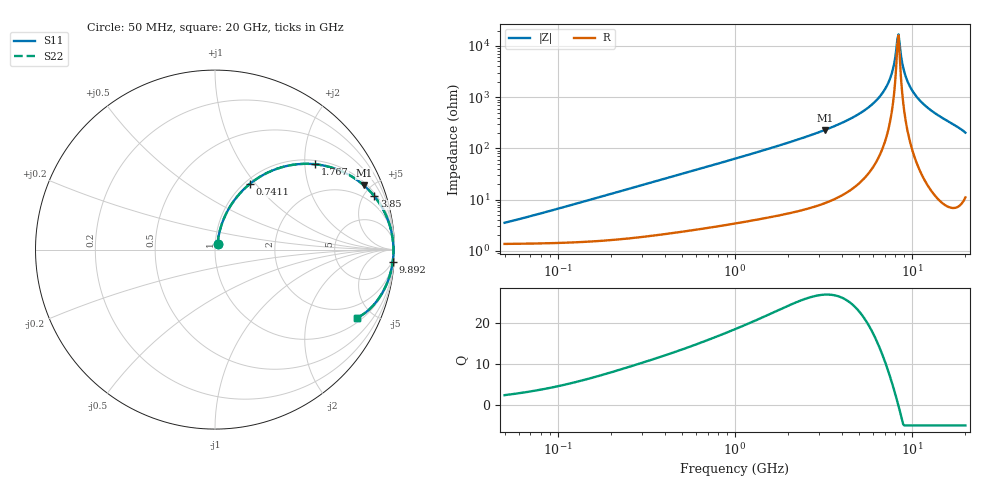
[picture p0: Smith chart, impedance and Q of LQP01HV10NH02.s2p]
!Murata Part Number: LQP01HV10NH02
!These Parameters are Measured in Series Mode Connection
!  o--[Z]--o
!Port1  Port2
!  o-------o
!Freq. Start=50[MHz] Stop=20[GHz], 401[Steps]
# Hz S RI R 50
!Freq.(Hz) S11(Real) S11(Imag) S21(Real) S21(Imag) S12(Real) S12(Imag) S22(Real) S22(Imag)
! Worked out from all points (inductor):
!   401 points, 50 MHz to 20 GHz, reference 50 ohm
!   read as one part in series: L = 10.3 nH near 63.54 MHz
!   highest Q = 26.9 at 3.217 GHz (marker M1), where L = 11.3 nH
!   self-resonance near 8.265 GHz
!   S11 on the Smith chart (normalised r, x): 50 MHz: 1.03, +0.06; 741.1 MHz: 1.06, +0.93; 1.767 GHz: 1.10, +2.26; 3.85 GHz: 1.22, +5.90; 9.892 GHz: 3, -29; 20 GHz: 1.22, -4.05
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5e7  0.0144 0.0315  0.9856 -0.0315  0.9856 -0.0315  0.0144 0.0315
1.364002e8  0.0219 0.0848  0.9781 -0.0848  0.9781 -0.0848  0.0219 0.0848
3.721004e8  0.0699 0.2155  0.9301 -0.2155  0.9301 -0.2155  0.0699 0.2155
7.411344e8  0.1931 0.3651  0.8069 -0.3651  0.8069 -0.3651  0.1931 0.3651
1e9  0.2932 0.4289  0.7068 -0.4289  0.7068 -0.4289  0.2932 0.4289
1.766834e9  0.5587 0.4754  0.4413 -0.4754  0.4413 -0.4754  0.5587 0.4754
2.728004e9  0.766 0.4049  0.234 -0.4049  0.234 -0.4049  0.766 0.4049
3.216634e9  0.8303 0.3572  0.1697 -0.3572  0.1697 -0.3572  0.8303 0.3572
3.850025e9  0.8881 0.2969  0.1119 -0.2969  0.1119 -0.2969  0.8881 0.2969
4.89267e9  0.9445 0.2086  0.0555 -0.2086  0.0555 -0.2086  0.9445 0.2086
5.944466e9  0.974 0.1337  0.026 -0.1337  0.026 -0.1337  0.974 0.1337
6.802353e9  0.9866 0.0811  0.0134 -0.0811  0.0134 -0.0811  0.9866 0.0811
7.442007e9  0.9917 0.0457  0.00834 -0.0457  0.00834 -0.0457  0.9917 0.0457
7.784049e9  0.9932 0.028  0.00679 -0.028  0.00679 -0.028  0.9932 0.028
8.141811e9  0.9941 0.0102  0.0059 -0.0102  0.0059 -0.0102  0.9941 0.0102
8.389408e9  0.9943 -0.00168  0.00567 0.00168  0.00567 0.00168  0.9943 -0.00168
8.516016e9  0.9943 -0.00764  0.00567 0.00764  0.00567 0.00764  0.9943 -0.00764
9.041845e9  0.9936 -0.0315  0.00639 0.0315  0.00639 0.0315  0.9936 -0.0315
9.892087e9  0.9902 -0.0677  0.00975 0.0677  0.00975 0.0677  0.9902 -0.0677
1.098561e10  0.9827 -0.1103  0.0173 0.1103  0.0173 0.1103  0.9827 -0.1103
1.257102e10  0.9666 -0.1661  0.0334 0.1661  0.0334 0.1661  0.9666 -0.1661
2e10  0.7918 -0.3797  0.2082 0.3797  0.2082 0.3797  0.7918 -0.3797
